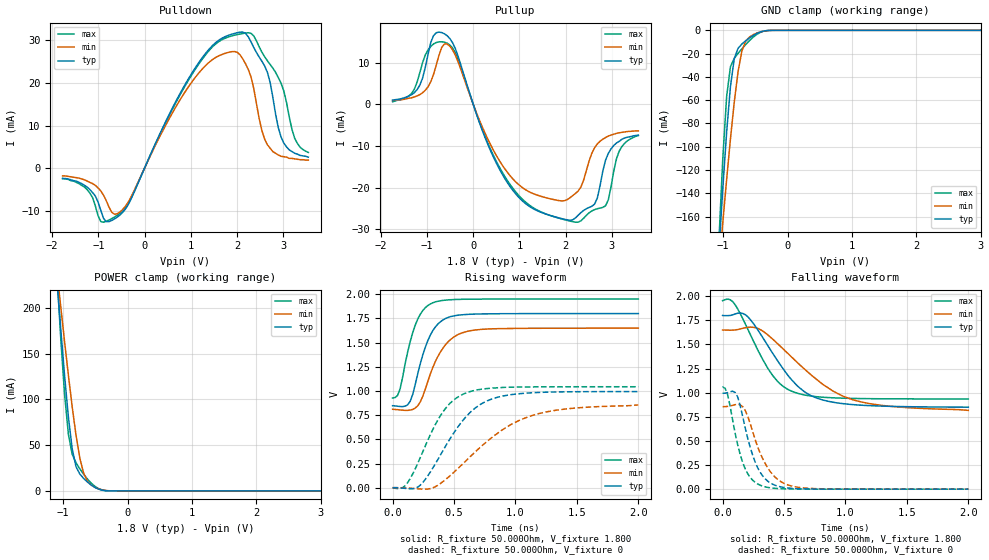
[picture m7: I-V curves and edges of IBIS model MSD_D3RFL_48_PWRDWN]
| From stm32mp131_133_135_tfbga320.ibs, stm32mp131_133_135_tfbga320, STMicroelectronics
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[Model] MSD_D3RFL_48_PWRDWN
Model_type   I/O
C_comp 2.550pF   2.464pF   2.678pF
Vinh = 1.440V
Vinl = 360.000mV
Vmeas = 900.000mV
Vref = 900.000mV
[Model Spec]
Vinh   1.440V   1.365V   1.515V
Vinl   360.000mV   285.000mV   435.000mV
Vmeas   900.000mV   825.000mV   975.000mV
Vref   900.000mV   825.000mV   975.000mV
[Temperature Range]   25.000   125.000   -40.000
[Voltage Range]   1.800V   1.650V   1.950V
[GND Clamp Reference]   0.00V   0.00V   0.00V
[Pulldown Reference]   0.00V   0.00V   0.00V
[POWER Clamp Reference]   1.800V   1.650V   1.950V
[Pullup Reference]   1.800V   1.650V   1.950V
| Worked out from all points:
|   slope of the pulldown table from 0 to 0.27 V, typ, clamps not added: 41 ohm
|   slope of the pullup table from 0 to 0.27 V, typ, clamps not added: 32.3 ohm
|   GND clamp passes 1 mA (typ) near -0.40 V on its own axis
|   POWER clamp passes 1 mA (typ) near -0.40 V on its own axis
|   rising waveform, R_fixture 50.000Ohm, V_fixture 1.800: 20-80 % time 142ps typ, 179ps min, 126ps max; typ from 0.848 V to 1.8 V
|   rising waveform, R_fixture 50.000Ohm, V_fixture 0: 20-80 % time 321ps typ, 504ps min, 252ps max; typ from 0.001 V to 0.994 V
|   falling waveform, R_fixture 50.000Ohm, V_fixture 1.800: 20-80 % time 330ps typ, 481ps min, 262ps max; typ from 1.8 V to 0.85 V
|   falling waveform, R_fixture 50.000Ohm, V_fixture 0: 20-80 % time 140ps typ, 171ps min, 120ps max; typ from 0.994 V to 0 V
[GND Clamp]
-1.773V   -892.4mA   -683.3mA   -1.196A
-1.064V   -188.1mA   -202.5mA   -178.5mA
-1.005V   -135.3mA   -164.6mA   -109.5mA
-945.5mV  -87.16mA   -127.9mA   -56.6mA
-886.4mV  -48.05mA   -93.1mA    -31.14mA
-827.3mV  -24.29mA   -61.54mA   -24.05mA
-768.2mV  -15.45mA   -35.41mA   -19.8mA
-709.1mV  -11.76mA   -17.8mA    -15.89mA
-650mV    -8.985mA   -9.267mA   -12.21mA
-531.8mV  -4.349mA   -3.679mA   -5.81mA
-295.4mV  -102.5uA   -159.7uA   -89.52uA
3.545V    35.5nA     528.3nA    5.672nA
[Power Clamp]
-1.745V   862.2mA    676.3mA    1.129A
-1.095V   229.4mA    238.8mA    234.5mA
-1.036V   175.7mA    200.4mA    165.4mA
-977.3mV  125.3mA    162.7mA    105mA
-918.2mV  80.5mA     126.2mA    61.63mA
-859.1mV  45.79mA    91.68mA    40mA
-800mV    26.41mA    60.76mA    30.8mA
-740.9mV  18.45mA    35.84mA    24.13mA
-681.8mV  13.67mA    19.37mA    18.21mA
-504.5mV  3.741mA    3.845mA    4.895mA
-268.2mV  31.85uA    110.6uA    36.37uA
3.573V    -37.18nA   -641.8nA   -5.478nA
[Pulldown]
-1.773V   -2.4mA     -1.8mA     -2.4mA
-1.241V   -4.4mA     -3mA       -5mA
-945.5mV  -9.88mA    -5.3mA     -12.48mA
-531.8mV  -10.94mA   -10.23mA   -10.54mA
1.064V    22.92mA    20.76mA    22.58mA
1.595V    29.86mA    26.24mA    29.55mA
2.068V    31.84mA    26.53mA    31.41mA
2.305V    29.56mA    21.37mA    31.56mA
2.659V    22.44mA    5.5mA      25.15mA
3.014V    5.9mA      2.7mA      18.1mA
3.25V     3.5mA      2.2mA      7mA
3.545V    2.6mA      1.9mA      3.7mA
[Pullup]
-1.745V   1mA        900uA      600uA
-1.332V   2.3mA      1.554mA    2.623mA
-1.036V   8.9mA      3.377mA    11.85mA
-859.1mV  16.47mA    7.15mA     14.48mA
-622.7mV  16.92mA    14.48mA    14.9mA
-386.4mV  13.35mA    11.77mA    12.34mA
795.5mV   -19.73mA   -17.13mA   -19.24mA
2.214V    -27.27mA   -21.4mA    -28.31mA
2.686V    -22.49mA   -9.523mA   -25.08mA
2.982V    -10.7mA    -7.392mA   -19.85mA
3.159V    -8.9mA     -6.846mA   -11.25mA
3.573V    -7.4mA     -6.4mA     -7.508mA
[Ramp]
R_load=50.000Ohm
dV/dt_r   583.770mV/232.000ps  505.679mV/337.000ps  617.730mV/189.500ps
dV/dt_f   583.678mV/235.500ps  504.320mV/323.000ps  617.730mV/191.000ps
[Rising waveform]
R_fixture=50.000Ohm
V_fixture=1.800
V_fixture_min=1.650
V_fixture_max=1.950
0s        848.1mV    811.1mV    928mV
41ps      842.9mV    807.1mV    954.7mV
62ps      839.8mV    804.3mV    1.025V
143ps     892.8mV    802.7mV    1.508V
225ps     1.28V      886.5mV    1.792V
286ps     1.518V     1.095V     1.882V
327ps     1.623V     1.242V     1.911V
450ps     1.759V     1.506V     1.941V
633ps     1.793V     1.623V     1.949V
2ns       1.8V       1.65V      1.95V
[Rising waveform]
R_fixture=50.000Ohm
V_fixture=0
0s        1.086mV    1.1mV      -2.413mV
103ps     -6.168mV   -1.13mV    22.13mV
225ps     26.7mV     -12.31mV   310.6mV
327ps     202.8mV    -987.9uV   600.4mV
409ps     381.7mV    62.53mV    782.2mV
572ps     695.2mV    247.8mV    966.6mV
776ps     901.4mV    486.1mV    1.026V
1.103ns   979.1mV    733.4mV    1.042V
1.409ns   991.6mV    814.3mV    1.043V
2ns       994.1mV    856.2mV    1.044V
[Falling waveform]
R_fixture=50.000Ohm
V_fixture=1.800
V_fixture_min=1.650
V_fixture_max=1.950
0s        1.8V       1.649V     1.953V
82ps      1.806V     1.648V     1.944V
205ps     1.787V     1.677V     1.659V
307ps     1.611V     1.654V     1.392V
409ps     1.406V     1.554V     1.176V
572ps     1.12V      1.357V     1.01V
756ps     949.3mV    1.147V     959.5mV
1.062ns   876mV      925.4mV    940.4mV
1.369ns   858.2mV    858.4mV    936.1mV
2ns       849.7mV    816.3mV    934.7mV
[Falling waveform]
R_fixture=50.000Ohm
V_fixture=0
0s        993.5mV    854.5mV    1.057V
41ps      1V         857.3mV    980.5mV
82ps      1.015V     868.9mV    715.1mV
123ps     955mV      879.6mV    460.3mV
164ps     751.6mV    854.6mV    275.3mV
205ps     525.5mV    754.6mV    159.2mV
307ps     172.7mV    370.5mV    40.56mV
429ps     39.68mV    122.4mV    8.464mV
593ps     6.443mV    23.99mV    1.451mV
2ns       14.75uV    98.8uV     1.08uV
